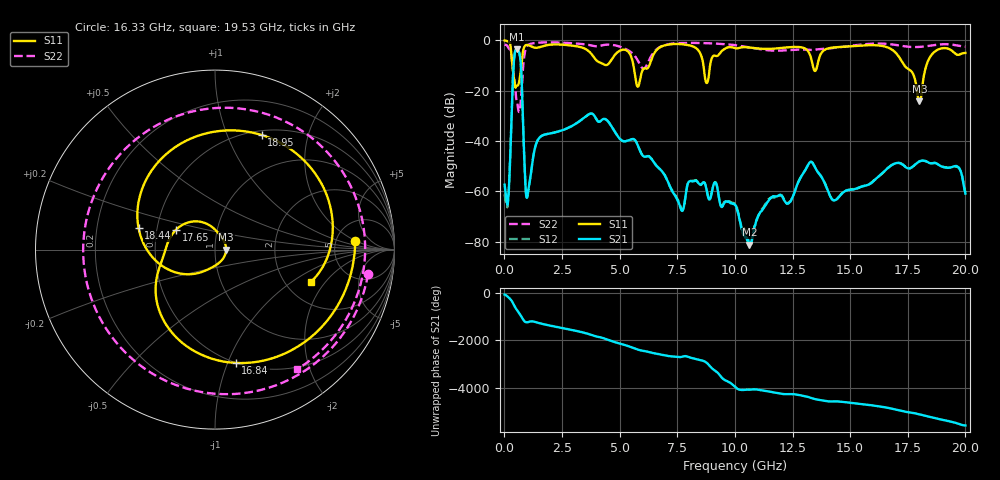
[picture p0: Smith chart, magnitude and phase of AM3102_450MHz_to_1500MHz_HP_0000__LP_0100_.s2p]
!Agilent Technologies,E8364B,MY43040894,A.07.50.67
!Agilent E8364B: A.07.50.67
!Date: Thursday, January 11, 2018 05:15:45
!Correction: S11(Full 2 Port(1,2))
!S21(Full 2 Port(1,2))
!S12(Full 2 Port(1,2))
!S22(Full 2 Port(1,2))
!S2P File: Measurements: S11, S21, S12, S22:
# Hz S  dB  R 50
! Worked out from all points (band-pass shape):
!   1601 points, 10 MHz to 20 GHz, reference 50 ohm
!   highest |S21| = -3.57 dB at 534.7 MHz (marker M1); lowest = -81.3 dB at 10.63 GHz (marker M2)
!   |S21| within 3 dB of the highest: 430.8 MHz to 681.6 MHz (250.8 MHz wide, 45.1 % of centre)
!   lowest |S11| = -24.2 dB at 18 GHz (marker M3), VSWR 1.13, Z = 56.6 + j0.0509 ohm
!   |S11| at or under -10 dB: 346.9 MHz to 738.8 MHz (391.9 MHz wide, 72.2 % of centre); 5.6 GHz to 6.287 GHz (687 MHz wide, 11.6 % of centre); 17.35 GHz to 18.31 GHz (951.7 MHz wide, 5.34 % of centre)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
!   |S22| runs from -28.5 to -0.8 dB; largest |S21 - S12| = 0.0024
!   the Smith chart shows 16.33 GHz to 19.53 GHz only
!   S11 on the Smith chart (normalised r, x): 16.33 GHz: 7.67, +1.96; 16.84 GHz: 0.50, -1.07; 17.65 GHz: 0.63, +0.15; 18.44 GHz: 0.39, +0.12; 18.95 GHz: 0.55, +1.34; 19.53 GHz: 2.72, -1.44
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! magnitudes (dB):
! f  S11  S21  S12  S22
! 10 MHz  0.0  -57.3  -61.2  -1.7
! 172.4 MHz  -0.6  -62.6  -63.2  -3.0
! 534.7 MHz  -18.1  -3.6  -3.6  -24.1
! 697.2 MHz  -13.2  -7.7  -7.7  -25.9
! 997 MHz  -1.9  -62.0  -62.3  -2.1
! 1.509 GHz  -2.8  -38.8  -38.8  -0.9
! 3.346 GHz  -2.8  -31.5  -31.5  -1.4
! 5.795 GHz  -18.4  -41.9  -41.9  -8.1
! 6.682 GHz  -3.2  -50.6  -50.6  -3.0
! 10.01 GHz  -3.1  -65.4  -64.9  -1.9
! 10.63 GHz  -2.9  -81.3  -81.7  -2.8
! 13.34 GHz  -8.4  -48.4  -48.3  -3.8
! 14.3 GHz  -2.8  -63.6  -63.6  -3.0
! 16.33 GHz  -2.1  -53.4  -53.4  -1.3
! 16.68 GHz  -3.0  -50.5  -50.4  -1.5
! 16.84 GHz  -3.8  -49.4  -49.4  -1.6
! 17.65 GHz  -12.2  -50.6  -50.6  -2.6
! 18 GHz  -24.2  -48.1  -48.1  -2.6
! 18.44 GHz  -7.1  -48.8  -48.8  -2.2
! 18.95 GHz  -3.2  -50.1  -50.0  -1.6
! 19.53 GHz  -5.0  -50.0  -50.2  -1.9
! 20 GHz  -5.0  -60.9  -60.5  -2.6
